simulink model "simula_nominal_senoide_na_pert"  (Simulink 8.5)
settings: Solver=ode45  StartTime=0.0  StopTime=tf  RelTol=1e-3
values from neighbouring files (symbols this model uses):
  denK = [1/6 1]    [princi_JL_incerto_prefilt_2a_ordem.m]
  knom = r*kT/Ra/Jeq    [princi_JL_incerto_prefilt_2a_ordem.m]
  numK = 2.5    [princi_JL_incerto_prefilt_2a_ordem.m]
  pnom = feq/Jeq    [princi_JL_incerto_prefilt_2a_ordem.m]
undefined symbols (not defined in the file or in its folder): w0_pert

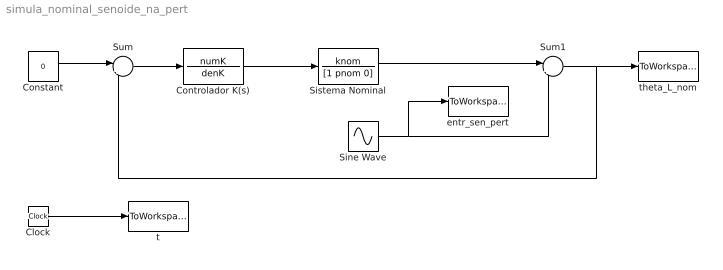
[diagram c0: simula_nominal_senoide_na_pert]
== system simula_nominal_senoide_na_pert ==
  Clock : Clock
  Constant : Constant  Value=0
  Controlador K(s) : TransferFcn  Numerator=numK  Denominator=denK
  Sine Wave : Sin  Frequency=w0_pert  SampleTime=0
  Sistema Nominal : TransferFcn  Numerator=knom  Denominator=[1 pnom 0]
  Sum : Sum  Inputs=|+-
  Sum1 : Sum  Inputs=|++
  entr_sen_pert : ToWorkspace  VariableName=entr_sen_pert  SampleTime=-1
  t : ToWorkspace  VariableName=t  SampleTime=-1
  theta_L_nom : ToWorkspace  VariableName=theta_L_nom  SampleTime=-1
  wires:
  Sum/1 -> Controlador K(s)/1
  Clock/1 -> t/1
  Controlador K(s)/1 -> Sistema Nominal/1
  Sine Wave/1 -> Sum1/2, entr_sen_pert/1
  Sistema Nominal/1 -> Sum1/1
  Sum1/1 -> Sum/2, theta_L_nom/1
  Constant/1 -> Sum/1
